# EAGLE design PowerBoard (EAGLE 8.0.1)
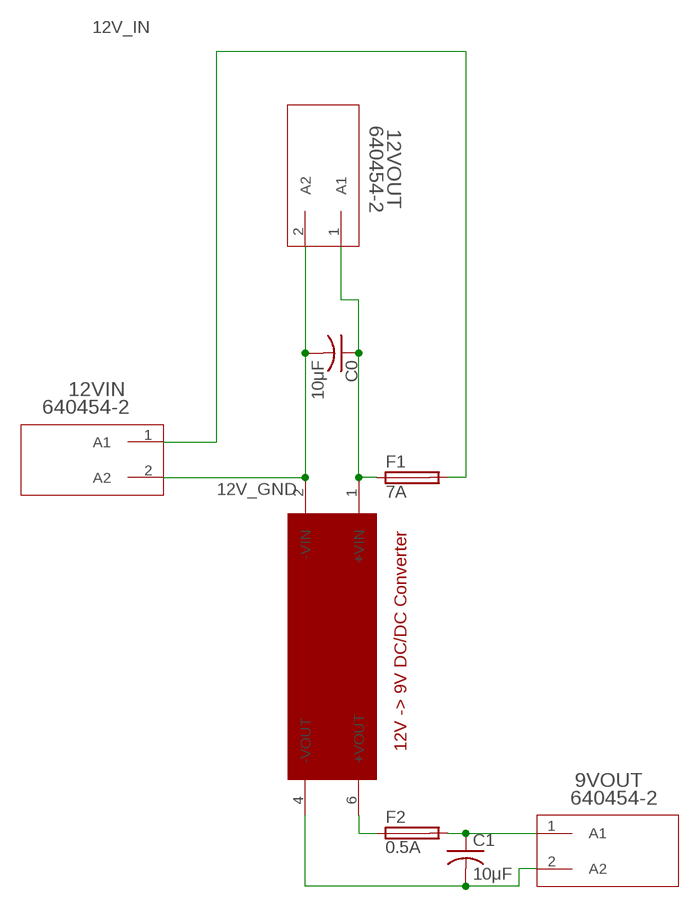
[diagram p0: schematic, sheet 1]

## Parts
9VOUT  640454-2  [640454-2]
12VIN  640454-2  [640454-2]
12VOUT  640454-2  [640454-2]
C0  C_10μF  [C_13MM]
C1  C_10μF  [C_13MM]
F1  7A  LITTLEFUSE  [LITTLEFUSE]
F2  0.5A  LITTLEFUSE  [LITTLEFUSE]
U$1  IR1209SA  [IR1209SA]

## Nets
9V: F2.1 U$1.6(+VOUT)
9V_GND: 9VOUT.2(A2) C1.- U$1.4(-VOUT)
9V_OUT: 9VOUT.1(A1) C1.+ F2.2
12V_GND: 12VIN.2(A2) 12VOUT.2(A2) C0.- U$1.2(-VIN)
12V_IN: 12VIN.1(A1) F1.2
12V_OUT: 12VOUT.1(A1) C0.+ F1.1 U$1.1(+VIN)

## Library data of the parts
9VOUT 12VIN 12VOUT = mta:640454-2; MANUFACTURER_PART_NUMBER: 6404542; VENDOR: Tyco Electronics
C0 C1 = ieee:C_10μF
F1 F2 = fuse:LITTLEFUSE: LITTLEFUSE; OC_FARNELL: unknown; OC_NEWARK: unknown
U$1 = xppower:IR1209SA

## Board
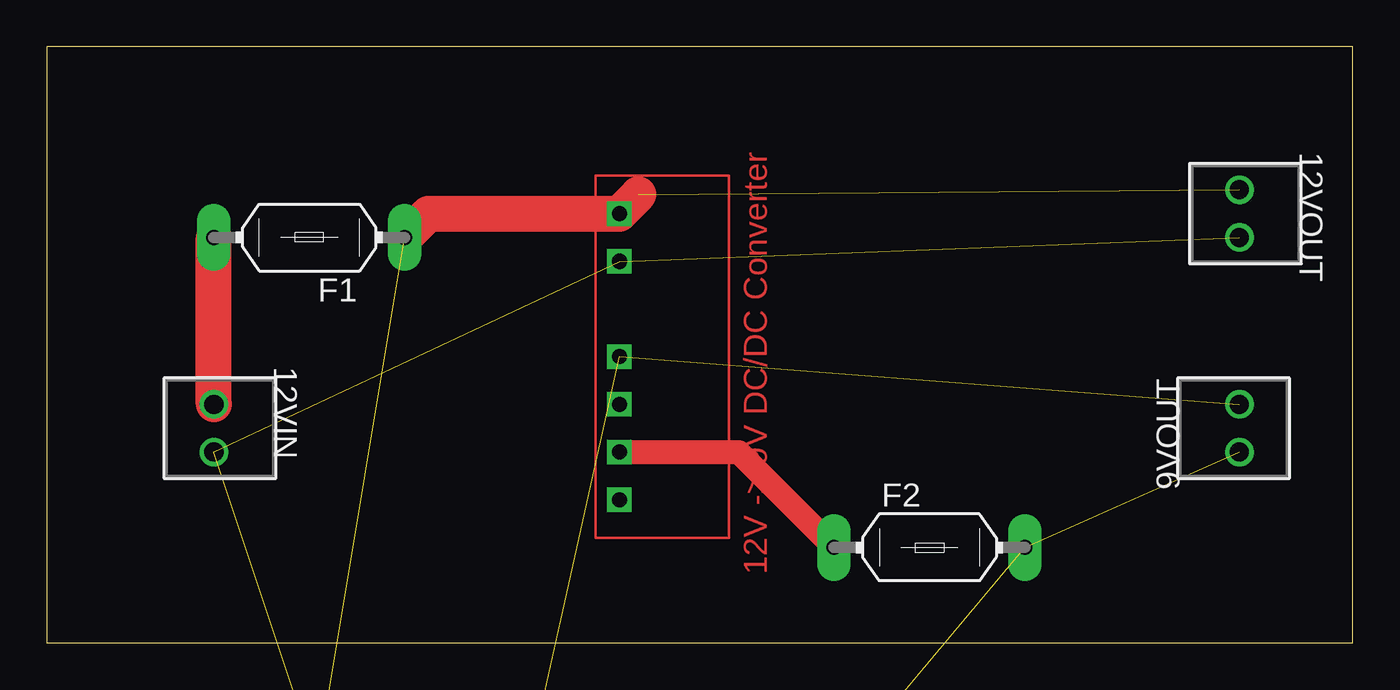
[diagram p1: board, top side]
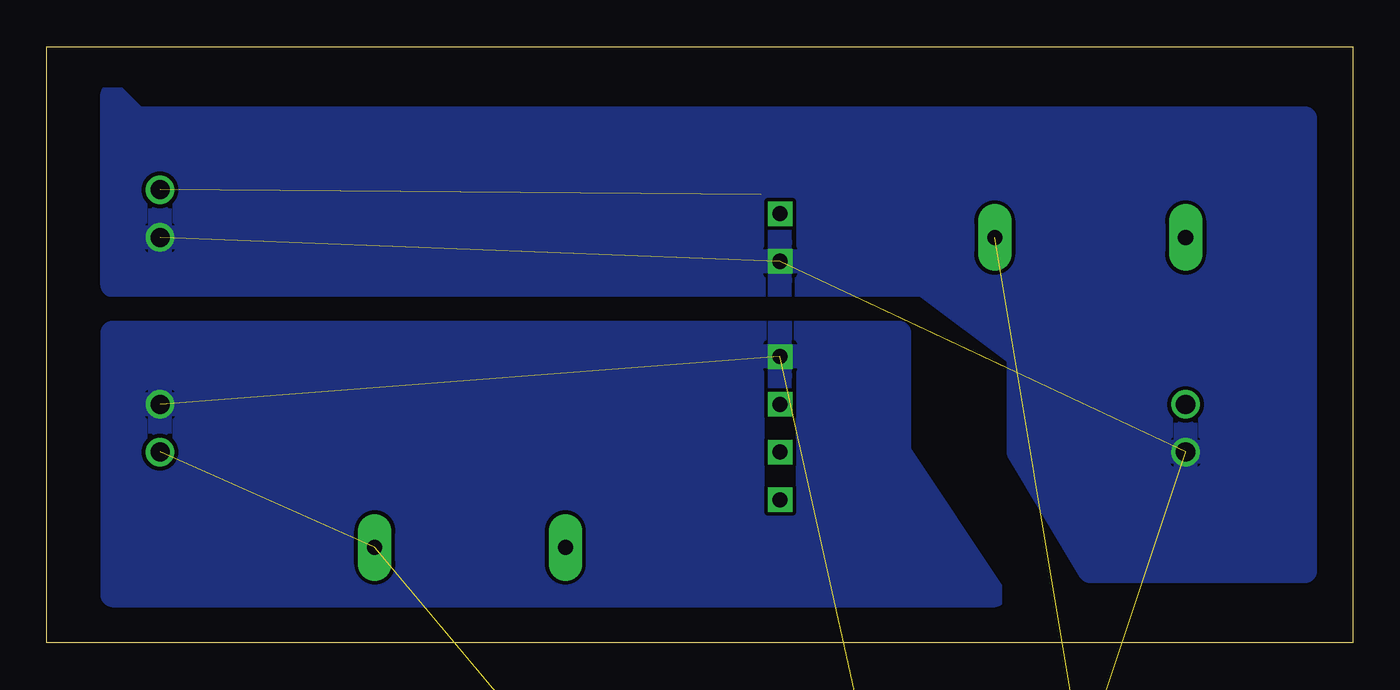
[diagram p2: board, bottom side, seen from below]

Size 69.52 x 31.74 mm. Coordinates in mm from the lower left corner, seen from the top.
Outline: 0,0 69.52,0 69.52,31.74 0,31.74 0,0
Copper layers (1*16): Top 0.035mm / dielectric 1.5mm / Bottom 0.035mm
Design rules "default": minimum track width 10mil, minimum drill 24mil, track to track 8mil, track to pad 8mil, pad to pad 8mil, via to via 8mil, smd to smd 8mil, copper to edge 40mil, drill to drill 8mil, minimum pad ring 10mil, minimum via ring 8mil, stop-mask expansion 4mil, vias tented up to drill 0mil, thermal gap 10mil

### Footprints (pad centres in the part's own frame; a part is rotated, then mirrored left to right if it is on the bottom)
640454-2 = drill 1.016 pad 1.524: 1 -2.54,0; 2 0,0
C_13MM = drill 1.016 pad 2.54: + -2.54,0 | drill 1.016 pad 2.54 octagon: - 2.54,0
LITTLEFUSE = drill 0.813 pad 1.778 long: 1 -5.08,0; 2 5.08,0
IR1209SA = drill 0.8 square: 1 -7.62,0; 2 -5.08,0; 4 0,0; 5 2.54,0; 6 5.08,0; 7 7.62,0

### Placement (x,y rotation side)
9VOUT  63.5,12.7 90 top
12VIN  8.89,10.16 270 top
12VOUT  63.5,21.59 270 top
C0  not placed on the board
C1  not placed on the board
F1  13.97,21.59 180 top
F2  46.99,5.08 0 top
U$1  30.48,15.24 270 top

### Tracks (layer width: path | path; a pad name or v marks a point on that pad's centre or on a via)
9V
  Top 1.27: U$1.6 36.83,10.16 F2.1
9V_GND  (2 unrouted)
  pour Bottom: 24.13,16.51 66.04,16.51 66.04,2.54 19.05,2.54 24.13,10.16
9V_OUT  (2 unrouted)
12V_GND  (3 unrouted)
  pour Bottom: 2.54,3.81 13.97,3.81 17.78,10.16 17.78,15.24 22.86,19.05 66.04,19.05 66.04,29.21 64.77,27.94 2.54,27.94
12V_IN
  Top 1.905: 12VIN.1 F1.2
12V_OUT  (2 unrouted)
  Top 1.905: F1.1 20.32,22.86 U$1.1 31.5,23.88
